{attribute 'call_after_init'}
FUNCTION_BLOCK FB_IED_IED EXTENDS FB_AcsiCommonIntelligentElectronicDeviceClass
VAR_INPUT
	IEDLD1: FB_LD_IEDLD1 := (bLinkResult:=THIS^.AddLogicalDeviceToContainer(ipLogicalDevice:=IEDLD1));
END_VAR
VAR
END_VAR

END_FUNCTION_BLOCK
